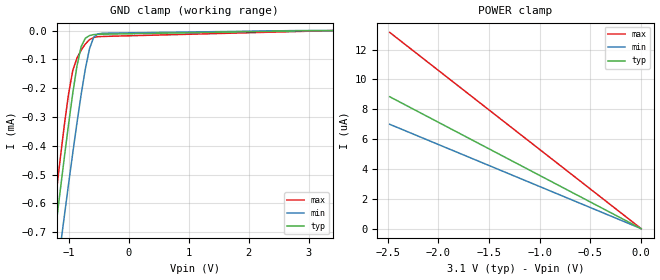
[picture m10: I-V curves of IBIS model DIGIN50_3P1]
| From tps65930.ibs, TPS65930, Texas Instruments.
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|   Model DIGIN50_3P1
[Model]   DIGIN50_3P1
Model_type   Input
Polarity   Non-Inverting
Vinl =   1.1935V
Vinh =   1.8135V
C_comp   0.3170pF   0.4534pF   0.3239pF
[Temperature Range]   25.0000   0.1250k   -40.0000
[Voltage Range]   3.1000V   2.7900V   3.4100V
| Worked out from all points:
|   GND clamp passes 1 mA (typ) near -1.39 V on its own axis
[GND_clamp]
| voltage   I(typ)   I(min)   I(max)
-3.1V     -4.031mA   -3.8mA     -4.266mA
-1.28V    -800.7uA   -984uA     -701.9uA
-1.21V    -678.6uA   -869.6uA   -573.2uA
-1.14V    -558.2uA   -756.3uA   -447.9uA
-1.07V    -440.4uA   -644.2uA   -328.3uA
-930mV    -218.6uA   -425.8uA   -139.4uA
-860mV    -123.6uA   -321.3uA   -95.68uA
-790mV    -55.64uA   -222.4uA   -68.12uA
-650mV    -17.23uA   -62.58uA   -31.52uA
-580mV    -14uA      -23.1uA    -23.66uA
-440mV    -12.65uA   -9.431uA   -20.48uA
3.41V     0A         0A         0A
[POWER_clamp]
| voltage   I(typ)   I(min)   I(max)
-2.48V    8.843uA    6.996uA    13.16uA
-1.56V    5.562uA    4.4uA      8.274uA
-920mV    3.28uA     2.595uA    4.879uA
0V        8.615pA    9.301pA    9.521pA
